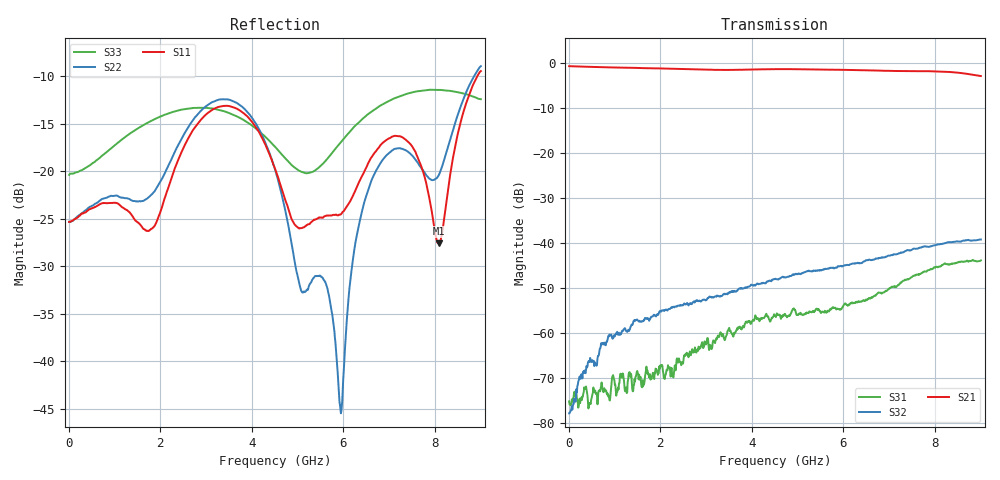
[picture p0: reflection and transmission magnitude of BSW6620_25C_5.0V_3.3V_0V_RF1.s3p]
!Agilent Technologies,N5230C,MY49001333,A.09.33.09
!Agilent N5230C: A.09.33.09
!Date: Monday, September 23, 2024 11:05:13
!Correction: S11(Full 3 Port(1,2,3))
!S12(Full 3 Port(1,2,3))
!S13(Full 3 Port(1,2,3))
!S21(Full 3 Port(1,2,3))
!S22(Full 3 Port(1,2,3))
!S23(Full 3 Port(1,2,3))
!S31(Full 3 Port(1,2,3))
!S32(Full 3 Port(1,2,3))
!S33(Full 3 Port(1,2,3))
!S3P File: Measurements: <S11,S12,S13>,
!<S21,S22,S23>,
!<S31,S32,S33>:
# Hz S  MA  R 50
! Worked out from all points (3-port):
!   901 points, 10 MHz to 9.01 GHz, reference 50 ohm
!   strongest paths, dB at 10 MHz, 2.26 GHz, 4.51 GHz, 6.76 GHz, 9.01 GHz:
!     S21: -0.6, -1.2, -1.3, -1.6, -2.8
!     S32: -77.8, -54.4, -47.9, -43.4, -39.1
!     S31: -75.2, -69.0, -56.1, -51.0, -43.8
!   lowest |S11| = -27.6 dB at 8.09 GHz (marker M1), VSWR 1.09, Z = 48.4 + j3.8 ohm
!   |S11| at or under -10 dB: start of sweep to 8.931 GHz
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1e7  0.05411 -2.9  0.9328 -2.8  8.21e-05 103.8
     0.9335 -2.7  0.0542 -2.2  0.0001984 -16.2
     0.0001747 12.0  0.0001285 32.5  0.09564 -4.6
1.4e9  0.05768 164.3  0.8948 -166.9  0.0002908 -70.9
       0.8947 -167.0  0.06983 -178.2  0.001248 -63.1
       0.000226 -62.0  0.001251 -60.5  0.1615 -156.5
2.23e9  0.08936 152.0  0.8757 94.6  0.0004133 -96.3
        0.876 94.5  0.1134 151.7  0.001899 -144.5
        0.0003286 -94.5  0.001905 -145.5  0.2033 131.1
3.02e9  0.2006 75.5  0.8535 1.8  0.0006881 173.5
        0.8535 1.5  0.2213 83.7  0.002223 126.4
        0.0008245 160.6  0.00238 131.9  0.2155 68.4
4.51e9  0.1032 -114.7  0.8642 -173.4  0.001645 -8.3
        0.8645 -173.6  0.1024 -66.4  0.004083 -25.4
        0.001562 -5.5  0.00401 -26.6  0.1346 -61.5
5.28e9  0.05334 77.3  0.8594 94.5  0.001817 -92.6
        0.8594 94.6  0.02564 -42.2  0.004868 -109.5
        0.001734 -94.9  0.004897 -109.2  0.09846 -166.3
6.03e9  0.06251 19.4  0.85 4.8  0.001876 -167.8
        0.8493 5.0  0.01067 114.2  0.005653 170.9
        0.002096 -166.8  0.005677 169.3  0.1501 96.4
6.9e9  0.1433 -35.8  0.833 -99.8  0.002971 111.6
       0.8294 -99.9  0.1179 -1.2  0.006951 77.5
       0.002856 112.4  0.006988 76.5  0.2277 18.5
8.09e9  0.04174 110.3  0.8138 114.1  0.005397 -29.8
        0.8149 113.7  0.09539 -55.8  0.008948 -50.8
        0.005489 -25.7  0.009731 -48.4  0.2679 -74.7
9.01e9  0.3368 -88.9  0.7181 0.7  0.006596 -143.3
        0.7249 -0.7  0.3573 -107.7  0.01101 -155.1
        0.006455 -142.4  0.01103 -150.3  0.2395 -147.2
